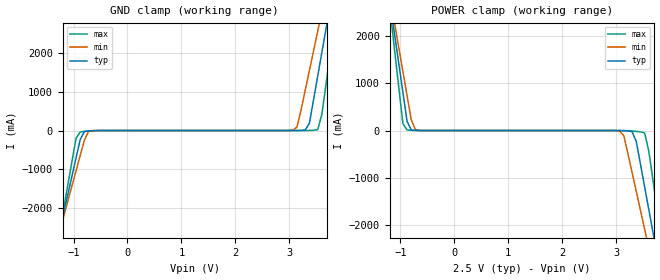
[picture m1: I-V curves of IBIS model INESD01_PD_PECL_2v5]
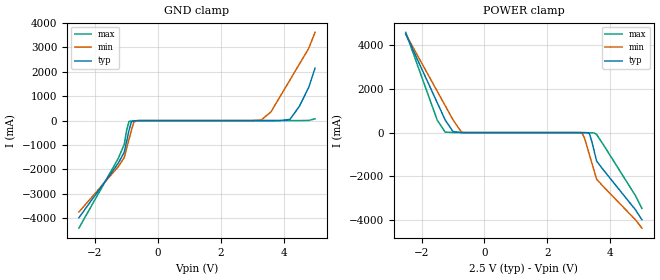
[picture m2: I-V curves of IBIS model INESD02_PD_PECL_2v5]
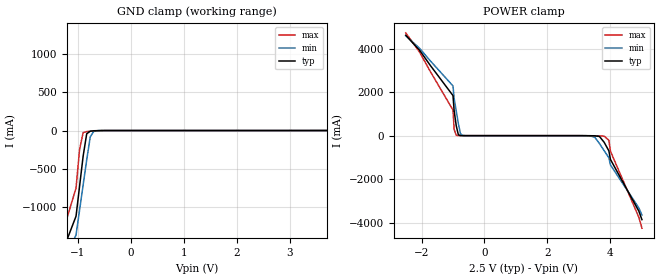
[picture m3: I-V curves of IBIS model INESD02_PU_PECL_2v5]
|   This file is an IBIS representation of the   |
|   Integrated Devices Technology, Inc.   |
|   ICS87332I-01   |
|   Divide by 2 Differential to ECL/LVPECL Generator   |
[IBIS Ver]   4.1
[File name]   87332i_01.ibs
[File Rev]   1.0
[Date]   19 Mar 2009 | Last modified
|   May 7 2003 | Generated
[Source]   Originated at Integrated Devices Technology, Inc.
[Disclaimer]
IDT hereby grants the user of this IBIS model a non-exclusive,
nontransferable license to use this IBIS model under the following terms.
Before using this IBIS model, the user should read this license.
If the user does not accept these terms,  the IBIS model should be
returned to IDT within 30 days.
   The user is granted this license only to use the IBIS model and
is not granted rights to sell, load, rent, lease or license the IBIS
model in whole or in part, or in modified form to anyone other than
user. User may modify the IBIS model to suit its specific
applications but rights to derivative works and such modifications
shall belong to IDT.
   This IBIS model is provided on an "AS IS" basis and IDT makes
absolutely no warranty with respect to the information contained
herein. IDT DISCLAIMS AND CUSTOMER WAIVES ALL WARRANTIES, EXPRESS
OR IMPLIED, INCLUDING WARRANTIES OF MERCHANTABILITY OR FITNESS FOR
A PARTICULAR PURPOSE. The entire risk as to quality and performance
is with the Customer. ACCORDINGLY, IN NO EVENT SHALL THE COMPANY BE
LIABLE FOR ANY DAMAGES, WHETHER IN CONTRACT OR TORT,INCLUDING ANY
LOST PROFITS OR OTHER INCIDENTAL, CONSEQUENTIAL, EXEMPLARY, OR
PUNITIVE DAMAGES ARISING OUT OF THE USE OR APPLICATION OF THE IBIS
model provided in this package. Further, IDT reserves the right to
make changes without notice to any product herein to improve
reliability, function, or design. IDT does not convey any license
under patent rights or any other intellectual property rights,
including those of third parties.
   IDT is not obligated to provide maintenance or support
for the licensed IBIS model.
[Copyright]   Copyright 2003 by Integrated Devices Technology, Inc.
[Component]   ICS87332I-01
[Manufacturer] Integrated Devices Technology, Inc.
[Package]
|SOIC 8 Lead
|   typ   min   max
R_pkg   57.05m   55.5m   58.6m
L_pkg   1.769nH   1.570nH   1.968nH
C_pkg   0.269pF   0.252pF   0.286pF
[Pin]   signal_name   model_name   R_pin   L_pin   C_pin
1   MR   INESD01_PD_PECL   58.6m   1.968n   0.286p
2   CLK   INESD02_PD_PECL   55.5m   1.570n   0.252p
3   nCLK   INESD02_PU_PECL   55.5m   1.570n   0.252p
4   nc   nc   56.6m   1.968n   0.286p
5   VEE   GND   58.6m   1.968n   0.286p
6   nQ   ONF01_HSTL01   55.5m   1.570n   0.252p
7   Q   ONF01_HSTL01   55.5m   1.570n   0.252p
8   VCC   POWER   56.6m   1.968n   0.286p
[Diff Pin]  inv_pin  vdiff tdelay_typ tdelay_min  tdelay_max
2   3   NA   0  0  0
7   6   NA   0  0  0
[Model Selector] INESD01_PD_PECL
INESD01_PD_PECL_2v5  Buffer selection for 2v5
INESD01_PD_PECL_3v3  Buffer selection for 3v3
[Model Selector] INESD02_PD_PECL
INESD02_PD_PECL_2v5  Buffer selection for 2v5
INESD02_PD_PECL_3v3  Buffer selection for 3v3
[Model Selector] INESD02_PU_PECL
INESD02_PU_PECL_2v5  Buffer selection for 2v5
INESD02_PU_PECL_3v3  Buffer selection for 3v3
[Model Selector] ONF01_HSTL01
ONF01_HSTL01_2v5  Buffer selection for 2v5
ONF01_HSTL01_3v3  Buffer selection for 3v3
| Models and submodels in the file (8): INESD01_PD_PECL_2v5 (Input), INESD02_PD_PECL_2v5 (Input), INESD02_PU_PECL_2v5 (Input), ONF01_HSTL01_2v5 (Output_ECL), INESD01_PD_PECL_3v3 (Input), INESD02_PD_PECL_3v3 (Input), INESD02_PU_PECL_3v3 (Input), ONF01_HSTL01_3v3 (Output_ECL)
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[Model] INESD01_PD_PECL_2v5
Model_type  Input
Polarity   Non-Inverting
Vinl = 0.9
Vinh = 1.6V
|   typ   min   max
C_comp   2pF   1.5pF   2.5pF
|   typ   min   max
[Voltage range]  2.5V   2.375V   2.625V
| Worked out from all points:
|   GND clamp passes 1 mA (typ) near -0.55 V on its own axis
|   POWER clamp passes 1 mA (typ) near -0.67 V on its own axis
[GND_clamp]
|Voltage   I(typ)   I(min)   I(max)
-2.5V     -10.33A    -9.044A    -12.47A
-1.263V   -2.632A    -2.639A    -2.655A
-953.6mV  -711.7mA   -1.044A    -200.4mA
-876.3mV  -232.7mA   -645.9mA   -36.86mA
-644.3mV  -3.696mA   -3.384mA   -8.124mA
3.067V    149.4uA    7.715mA    47.92uA
3.144V    502.3uA    86.83mA    64.06uA
3.376V    191.2mA    1.558A     2.431mA
3.531V    1.419A     2.581A     23.33mA
3.686V    2.649A     3.605A     1.215A
3.84V     3.882A     4.631A     2.791A
5V        13.16A     12.34A     14.65A
[POWER_clamp]
|Voltage   I(typ)   I(min)   I(max)
-2.5V     13.16A     11.51A     15.93A
-1.186V   2.649A     2.777A     2.489A
-1.108V   2.034A     2.265A     1.701A
-953.6mV  804mA      1.243A     144.3mA
-876.3mV  191.2mA    733.1mA    11.85mA
-644.3mV  502.3uA    1.889mA    389.3uA
3.067V    -1.226mA   -11.24mA   -226.8uA
3.299V    -24.5mA    -891.1mA   -10.73mA
3.531V    -1.191A    -2.086A    -51.9mA
3.686V    -2.151A    -2.885A    -1.049A
3.84V     -3.112A    -3.684A    -2.276A
5V        -10.33A    -9.692A    -11.48A
[Model] INESD02_PD_PECL_2v5
Model_type   Input
Polarity   Non-Inverting
Vinl = 0.8V
Vinh = 2.0V
|   typ   min   max
C_comp   2pF   1.5pF   2.5pF
|   typ   min   max
[Voltage range]  2.5V   2.375V   2.625V
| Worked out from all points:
|   GND clamp passes 1 mA (typ) near -0.59 V on its own axis
|   POWER clamp passes 1 mA (typ) near -0.69 V on its own axis
[GND_clamp]
|Voltage   I(typ)   I(min)   I(max)
-2.5V     -3.983A    -3.749A    -4.408A
-1.25V    -1.747A    -1.889A    -1.551A
-1.061V   -1.3A      -1.517A    -979.1mA
-909.1mV  -407.1mA   -774.3mA   -35.24mA
-833.3mV  -48.47mA   -403.4mA   -14.47mA
-757.6mV  -7.272mA   -70.21mA   -9.677mA
-681.8mV  -2.863mA   -7.067mA   -5.73mA
3.3V      167.2uA    32.81mA    49.66uA
3.6V      586.4uA    357.8mA    70.1uA
4.2V      47.81mA    1.661A     649.6uA
4.8V      1.366A     2.965A     5.596mA
5V        2.15A      3.618A     75.79mA
[POWER_clamp]
|Voltage   I(typ)   I(min)   I(max)
-2.5V     4.503A     4.499A     4.579A
-1.5V     1.366A     1.889A     566.5mA
-1.25V    582.4mA    1.237A     24.21mA
-1V       47.81mA    585.7mA    3.595mA
-681.8mV  586.4uA    6.896mA    416.8uA
3.03V     -323.1uA   -3.378mA   -47.98uA
3.106V    -1.127mA   -30.71mA   -286.5uA
3.182V    -2.863mA   -273.7mA   -1.276mA
3.333V    -48.47mA   -1.016A    -7.036mA
3.561V    -1.3A      -2.13A     -81.94mA
4.8V      -3.536A    -3.991A    -2.894A
5V        -3.983A    -4.363A    -3.465A
[Model] INESD02_PU_PECL_2v5
Model_type   Input
Polarity   Non-Inverting
Vinl = .8V
Vinh =  2V
|   typ   min   max
C_comp   2pF   1.5pF   2.5pF
|   typ   min   max
[Voltage range]  2.5V   2.375V   2.625V
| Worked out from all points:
|   GND clamp passes 1 mA (typ) near -0.59 V on its own axis
|   POWER clamp passes 1 mA (typ) near -0.70 V on its own axis
[GND_clamp]
|Voltage   I(typ)   I(min)   I(max)
-2.5V     -3.894A    -3.674A    -4.294A
-1.25V    -1.521A    -1.7A      -1.261A
-1.031V   -1.125A    -1.372A    -755.3mA
-896.9mV  -335.4mA   -714.7mA   -27.06mA
-695.9mV  -3.401mA   -10.7mA    -6.467mA
3.995V    711.6uA    10.32mA    481.3uA
4.062V    4.029mA    88.04mA    1.401mA
4.129V    40.44mA    547.3mA    3.341mA
4.196V    445.8mA    1.124A     14.79mA
4.263V    1.139A     1.7A       275.9mA
4.5V      1.832A     2.277A     1.163A
5V        3.219A     3.431A     2.937A
[POWER_clamp]
|Voltage   I(typ)   I(min)   I(max)
-2.5V     4.617A     4.594A     4.726A
-1V       1.842A     2.286A     1.176A
-963.9mV  1.149A     1.709A     289.6mA
-896.9mV  456.4mA    1.132A     15.33mA
-829.9mV  42.02mA    556.1mA    3.389mA
-762.9mV  4.159mA    91.01mA    1.421mA
-695.9mV  727.9uA    10.67mA    490.4uA
3.35V     -3.204mA   -9.193mA   -6.2mA
3.8V      -305mA     -689.5mA   -24.7mA
3.95V     -699.9mA   -1.018A    -211mA
4V        -1.095A    -1.346A    -716.4mA
5V        -3.863A    -3.649A    -4.255A
